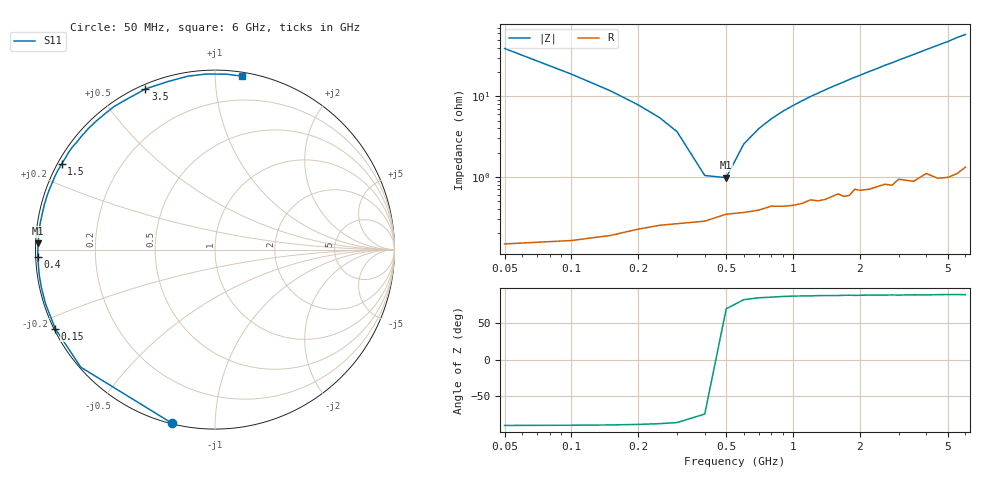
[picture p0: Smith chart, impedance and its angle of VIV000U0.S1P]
! Infineon Technologies  Discrete & RF Semiconductors
! BB 804
! Si Tuning Diode in SOT23
! VR = 0 V
! S-Parameters:  July  1999
# GHz  S  MA  R  50
!  f  S11
! GHz  MAG  ANG
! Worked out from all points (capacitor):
!   34 points, 50 MHz to 6 GHz, reference 50 ohm
!   read as one part to ground: C = 80.5 pF near 50 MHz
!   lowest |Z| = 979 mohm at 500 MHz (marker M1)
!   series resonance near 452.3 MHz, so ESL is about 1.5 nH
!   S11 on the Smith chart (normalised r, x): 50 MHz: 0.00, -0.78; 150 MHz: 0.00, -0.23; 400 MHz: 0.01, -0.02; 1.5 GHz: 0.01, +0.26; 3.5 GHz: 0.02, +0.66; 6 GHz: 0.03, +1.16
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0.05  0.9963 -104.0
0.1  0.9943 -138.8
0.15  0.9929 -153.7
0.2  0.9912 -162.2
0.25  0.9901 -167.6
0.3  0.9896 -171.7
0.4  0.9887 -177.7
0.5  0.9863 177.9
0.6  0.9856 174.2
0.8  0.9829 168.0
1  0.9828 162.6
1.2  0.9802 157.6
1.5  0.9788 150.7
1.6  0.9774 148.6
1.7  0.9792 146.5
1.8  0.9788 144.2
1.9  0.9751 142.1
2.2  0.9761 136.1
2.4  0.9749 132.4
2.6  0.974 128.4
2.8  0.9754 125.1
3  0.9718 121.4
3.5  0.9756 113.4
4  0.9723 105.7
4.5  0.978 98.9
5  0.9795 92.8
5.5  0.9796 86.3
6  0.9778 81.3
